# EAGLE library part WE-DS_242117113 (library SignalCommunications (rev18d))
WE-DS D-SUB-Filter Connectors Bent 90° Characteristics Standard type filtered with 1000 pF High attenuation of more than 40 dB @ 180 MHz Low size: 6.3 mm Rated voltage: 125 VDC Rated current @ 20 ºC: 5 A Withstand voltage: 250 VRMS Insulation resistance: min. 1000 MΩ Operating temperature: –55 ºC to +125 ºC Applications Filtering of interfaces External connection to -printer -sensor -display Details see: http://katalog.we-online.de/en/pbs/D-SUB-Filter Bent 90° Created on 2015-05-04 2015 (C) Wurth Elektronik
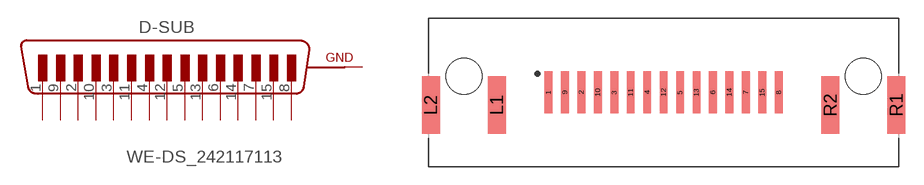
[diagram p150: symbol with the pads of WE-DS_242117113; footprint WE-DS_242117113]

Designator prefix D-SUB

## WE-DS_242117113 (WE-NUMBER: 242117113/15pins_male)  [WE-DS_242117113]
1  1  pas
2  2  pas
3  3  pas
4  4  pas
5  5  pas
6  6  pas
7  7  pas
8  8  pas
9  9  pas
10  10  pas
11  11  pas
12  12  pas
13  13  pas
14  14  pas
15  15  pas
L1  GND  pas
L2  GND  pas
R1  GND  pas
R2  GND  pas

## Footprint WE-DS_242117113 (pad centres in mm)
smd 0.65 x 3.5: 1 -9.59,0; 2 -6.85,0; 3 -4.11,0; 4 -1.37,0; 5 1.37,0; 6 4.11,0; 7 6.85,0; 8 9.59,0; 9 -8.22,0; 10 -5.48,0; 11 -2.74,0; 12 0,0; 13 2.74,0; 14 5.48,0; 15 8.22,0
smd 1.5 x 4.8: L1 -13.9,-1.05; L2 -19.4,-1.05; R1 19.4,-1.05; R2 13.9,-1.05
hole 3 at -16.65,1.35
hole 3 at 16.65,1.35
